(* Logix 5000 AddOnInstructionDefinition export SPEL_SpeedS; software revision 30.01 *)

ADD_ON_INSTRUCTION SPEL_ExecCmd   (* revision 1.2 *)
// Executes a command in the robot controller.  Normally this is called by higher level AOIs.
VAR_INPUT
   Start : BOOL; {required}
   MaxTime : DINT := 3000; {required}
END_VAR
VAR_OUTPUT
   InCycle : BOOL; {access Read Only, visible}
   Done : BOOL; {access Read Only, visible}
   Error : BOOL; {access Read Only, visible}
END_VAR
VAR_IN_OUT
   ExtInputs : AB:ETHERNET_MODULE_INT_128Bytes:I:0; {required}
        .DATA[0].0   // ExtCmdGet
        .DATA[0].1   // ExtRespSet
        .DATA[0].2   // ExtCmdResult
        .DATA[0].3   // ExtError
   ExtOutputs : AB:ETHERNET_MODULE_INT_128Bytes:O:0; {required}
        .DATA[0].0   // ExtCmdSet
        .DATA[0].1   // ExtRespGet
        .DATA[0].2   // ExtCmdReset
END_VAR
VAR_INPUT
   Cmd : INT; {required}
   CmdParam1 : INT; {required}
   CmdParam2 : INT; {required}
   CmdParam3 : INT; {required}
   CmdParam4 : INT; {required}
   CmdParam5 : INT; {required}
   CmdParam6 : INT; {required}
   CmdParam7 : INT; {required}
END_VAR
VAR_OUTPUT
   CmdEcho : INT; {access Read Only, visible}
   Resp1 : INT; {access Read Only, visible}
   Resp2 : INT; {access Read Only, visible}
   Resp3 : INT; {access Read Only, visible}
   Resp4 : INT; {access Read Only, visible}
   Resp5 : INT; {access Read Only, visible}
   Resp6 : INT; {access Read Only, visible}
   Resp7 : INT; {access Read Only, visible}
   ErrCode1 : INT; {access Read Only, visible}
   ErrCode2 : INT; {access Read Only, visible}
END_VAR
VAR
   ExtReset : BOOL; {access None}
   ExtError : BOOL; {access None}
   ExtCmdSet : BOOL; {access None}   // Cmd Ready
   ExtCmdGet : BOOL; {access None}   // Cmd Received
   CmdXferDone : BOOL; {access None}
   ExtRespSet : BOOL; {access None}   // Resp Ready
   RespXferDone : BOOL; {access None}
   ExtCmdResult : BOOL; {access None}   // Normal or Error?
   TmrCmdDataRdy : TIMER := (PRE := 5); {access None}
   OneShotDoneOff : BOOL; {access None}
   OneShotStart : BOOL; {access None}
   StartInit : BOOL; {access None}
   OneShotStartError : BOOL; {access None}
   TmrCycle : TIMER := (PRE := 5000); {access None}
   OneshotTmrPreset : BOOL; {access None}
   TmrCmdSet : TIMER := (PRE := 20); {access None}
   OnShotCmdDataXfer : BOOL; {access None}
   OneShotRespDataXfer : BOOL; {access None}
   OneShotDataRdy : BOOL; {access None}
   OtherCmdInCycle : BOOL; {access None}
   s : BOOL; {access None}
   OneShotUnsetCmdIncycle : BOOL; {access None}
   OneShotSetCmdIncycle : BOOL; {access None}
   OneShotSetOtherCmdInCycleError : BOOL; {access None}
   OneShotSetBit : BOOL; {access None}
   MaxTimeError : BOOL; {access None}
END_VAR

ROUTINE Logic   (* ladder *)
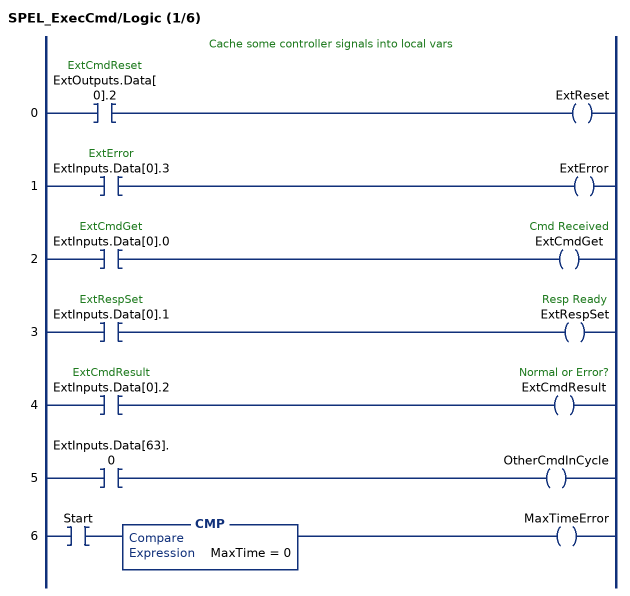
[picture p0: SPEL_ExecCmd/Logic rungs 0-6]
   // Cache some controller signals into local vars
   0: XIC(ExtOutputs.Data[0].2)OTE(ExtReset);
   1: XIC(ExtInputs.Data[0].3)OTE(ExtError);
   2: XIC(ExtInputs.Data[0].0)OTE(ExtCmdGet);
   3: XIC(ExtInputs.Data[0].1)OTE(ExtRespSet);
   4: XIC(ExtInputs.Data[0].2)OTE(ExtCmdResult);
   5: XIC(ExtInputs.Data[63].0)OTE(OtherCmdInCycle);
   6: XIC(Start)CMP(MaxTime = 0)OTE(MaxTimeError);
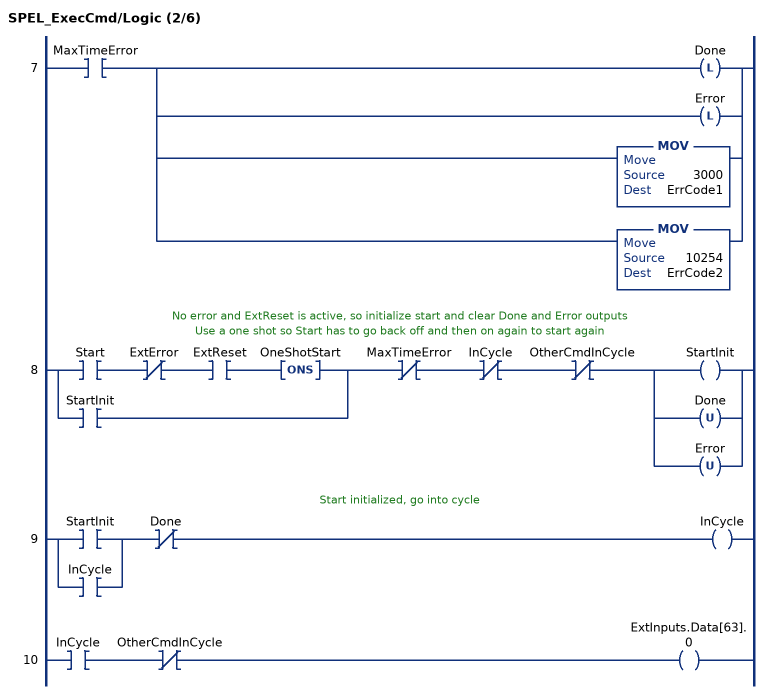
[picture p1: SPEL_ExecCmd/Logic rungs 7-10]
   7: XIC(MaxTimeError)[OTL(Done) ,OTL(Error) ,MOV(3000,ErrCode1) ,MOV(10254,ErrCode2) ];
   // No error and ExtReset is active, so initialize start and clear Done and Error outputs
   // Use a one shot so Start has to go back off and then on again to start again
   8: [XIC(Start) XIO(ExtError) XIC(ExtReset) ONS(OneShotStart) ,XIC(StartInit) ]XIO(MaxTimeError)XIO(InCycle)XIO(OtherCmdInCycle)[OTE(StartInit) ,OTU(Done) ,OTU(Error) ];
   // Start initialized, go into cycle
   9: [XIC(StartInit) ,XIC(InCycle) ]XIO(Done)OTE(InCycle);
   10: XIC(InCycle)XIO(OtherCmdInCycle)OTE(ExtInputs.Data[63].0);
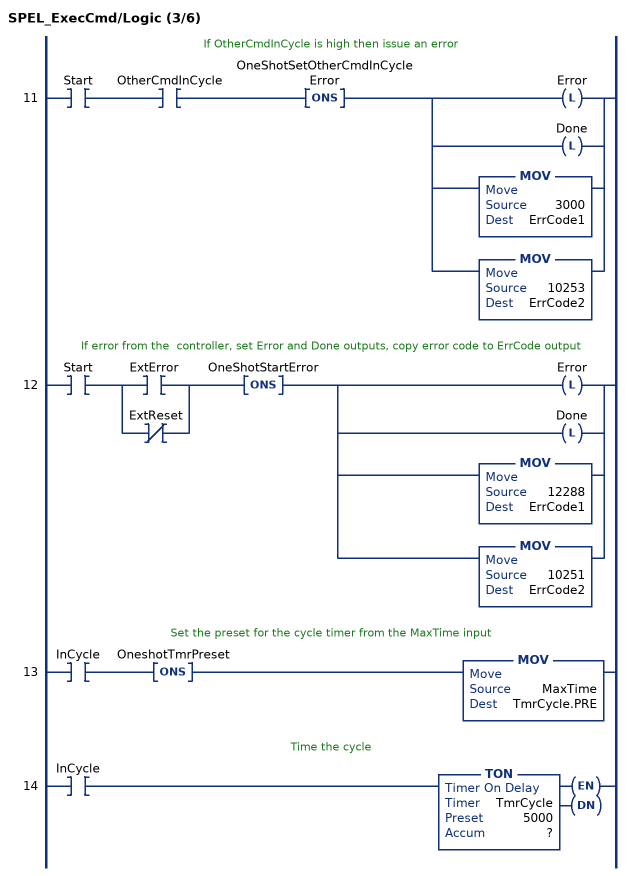
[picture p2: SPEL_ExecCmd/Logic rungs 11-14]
   // If OtherCmdInCycle is high then issue an error
   11: XIC(Start)XIC(OtherCmdInCycle)ONS(OneShotSetOtherCmdInCycleError)[OTL(Error) ,OTL(Done) ,MOV(3000,ErrCode1) ,MOV(10253,ErrCode2) ];
   // If error from the  controller, set Error and Done outputs, copy error code to ErrCode output
   12: XIC(Start)[XIC(ExtError) ,XIO(ExtReset) ]ONS(OneShotStartError)[OTL(Error) ,OTL(Done) ,MOV(12288,ErrCode1) ,MOV(10251,ErrCode2) ];
   // Set the preset for the cycle timer from the MaxTime input
   13: XIC(InCycle)ONS(OneshotTmrPreset)MOV(MaxTime,TmrCycle.PRE);
   // Time the cycle
   14: XIC(InCycle)TON(TmrCycle,?,?);
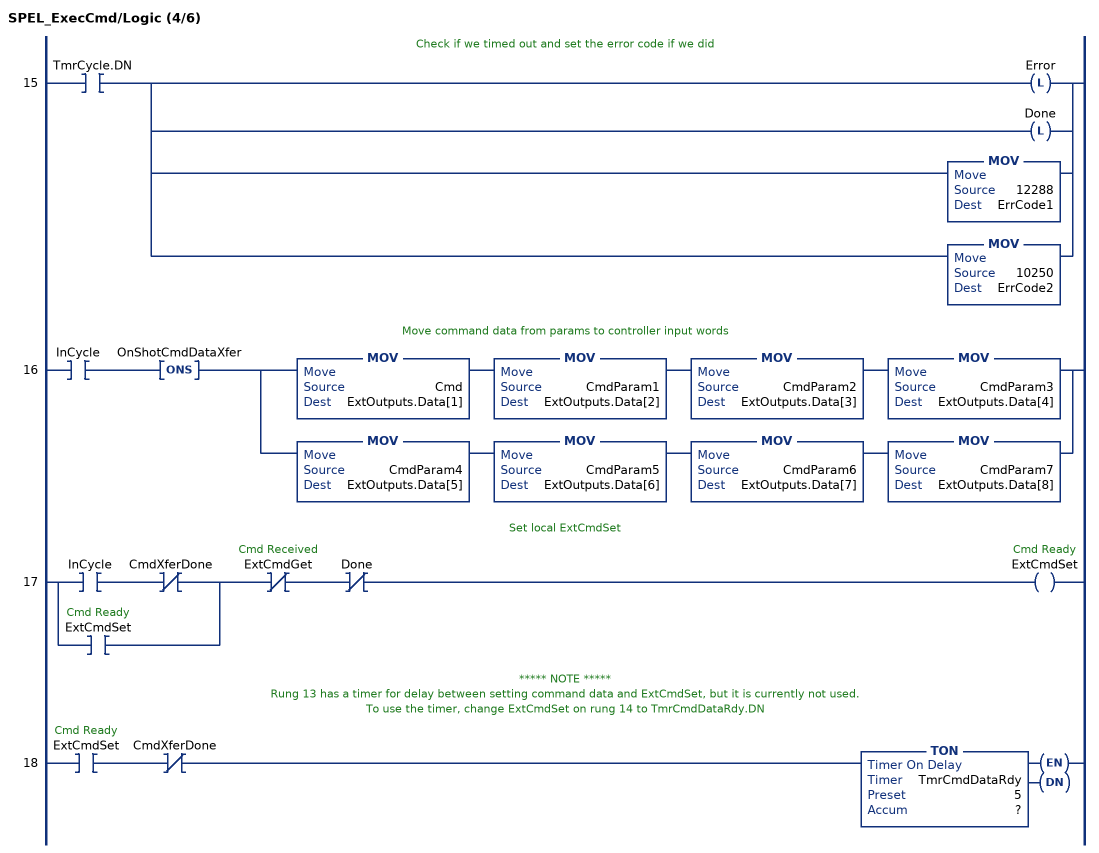
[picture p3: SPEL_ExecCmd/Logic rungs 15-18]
   // Check if we timed out and set the error code if we did
   15: XIC(TmrCycle.DN)[OTL(Error) ,OTL(Done) ,MOV(12288,ErrCode1) ,MOV(10250,ErrCode2) ];
   // Move command data from params to controller input words
   16: XIC(InCycle)ONS(OnShotCmdDataXfer)[MOV(Cmd,ExtOutputs.Data[1]) MOV(CmdParam1,ExtOutputs.Data[2]) MOV(CmdParam2,ExtOutputs.Data[3]) MOV(CmdParam3,ExtOutputs.Data[4]) ,MOV(CmdParam4,ExtOutputs.Data[5]) MOV(CmdParam5,ExtOutputs.Data[6]) MOV(CmdParam6,ExtOutputs.Data[7]) MOV(CmdParam7,ExtOutputs.Data[8]) ];
   // Set local ExtCmdSet
   17: [XIC(InCycle) XIO(CmdXferDone) ,XIC(ExtCmdSet) ]XIO(ExtCmdGet)XIO(Done)OTE(ExtCmdSet);
   // ***** NOTE *****
   // Rung 13 has a timer for delay between setting command data and ExtCmdSet, but it is currently not used.
   // To use the timer, change ExtCmdSet on rung 14 to TmrCmdDataRdy.DN
   18: XIC(ExtCmdSet)XIO(CmdXferDone)TON(TmrCmdDataRdy,?,?);
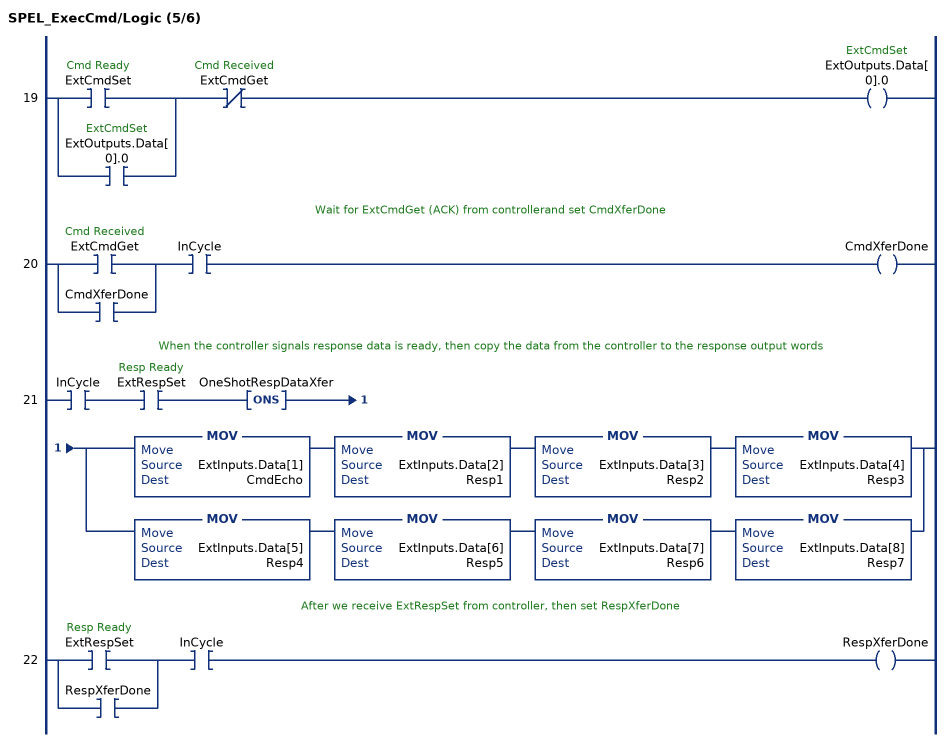
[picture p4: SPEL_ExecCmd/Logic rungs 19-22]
   19: [XIC(ExtCmdSet) ,XIC(ExtOutputs.Data[0].0) ]XIO(ExtCmdGet)OTE(ExtOutputs.Data[0].0);
   // Wait for ExtCmdGet (ACK) from controllerand set CmdXferDone
   20: [XIC(ExtCmdGet) ,XIC(CmdXferDone) ]XIC(InCycle)OTE(CmdXferDone);
   // When the controller signals response data is ready, then copy the data from the controller to the response output words
   21: XIC(InCycle)XIC(ExtRespSet)ONS(OneShotRespDataXfer)[MOV(ExtInputs.Data[1],CmdEcho) MOV(ExtInputs.Data[2],Resp1) MOV(ExtInputs.Data[3],Resp2) MOV(ExtInputs.Data[4],Resp3) ,MOV(ExtInputs.Data[5],Resp4) MOV(ExtInputs.Data[6],Resp5) MOV(ExtInputs.Data[7],Resp6) MOV(ExtInputs.Data[8],Resp7) ];
   // After we receive ExtRespSet from controller, then set RespXferDone
   22: [XIC(ExtRespSet) ,XIC(RespXferDone) ]XIC(InCycle)OTE(RespXferDone);
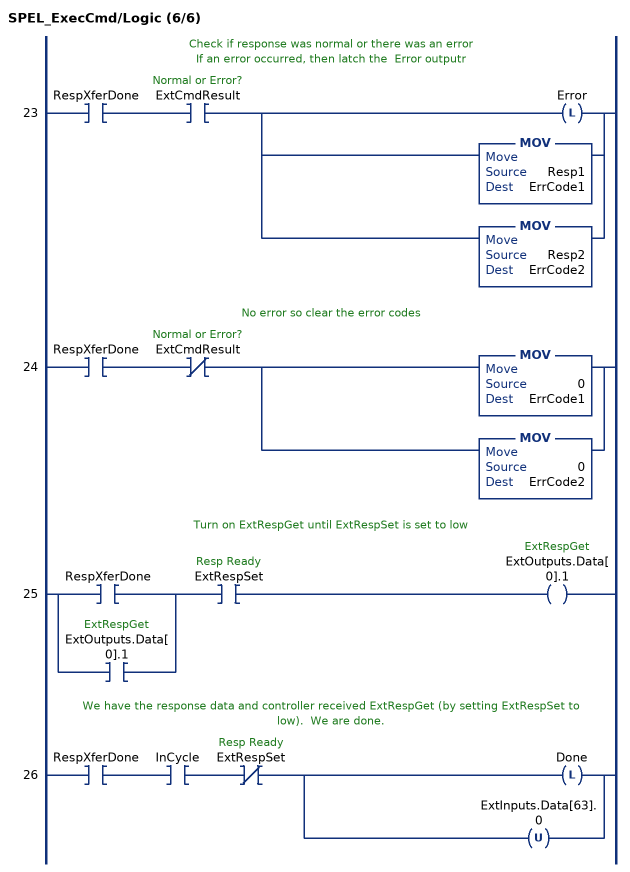
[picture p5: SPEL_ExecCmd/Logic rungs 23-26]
   // Check if response was normal or there was an error
   // If an error occurred, then latch the  Error outputr
   23: XIC(RespXferDone)XIC(ExtCmdResult)[OTL(Error) ,MOV(Resp1,ErrCode1) ,MOV(Resp2,ErrCode2) ];
   // No error so clear the error codes
   24: XIC(RespXferDone)XIO(ExtCmdResult)[MOV(0,ErrCode1) ,MOV(0,ErrCode2) ];
   // Turn on ExtRespGet until ExtRespSet is set to low
   25: [XIC(RespXferDone) ,XIC(ExtOutputs.Data[0].1) ]XIC(ExtRespSet)OTE(ExtOutputs.Data[0].1);
   // We have the response data and controller received ExtRespGet (by setting ExtRespSet to low).  We are done.
   26: XIC(RespXferDone)XIC(InCycle)XIO(ExtRespSet)[OTL(Done) ,OTU(ExtInputs.Data[63].0) ];
END_ROUTINE
END_ADD_ON_INSTRUCTION

ADD_ON_INSTRUCTION SPEL_SpeedS   (* revision 1.2, vendor SEIKO EPSON CORP. *)
// Sets the arm speed setting of CP motion. This will set the depart, and approach speed as well.
VAR_OUTPUT
   InCycle : BOOL; {access Read Only, visible}
   Done : BOOL; {access Read Only, visible}
   Error : BOOL; {access Read Only, visible}
END_VAR
VAR_INPUT
   Start : BOOL; {required}
   Speed : REAL; {required}
   ApproSpeed : REAL; {required}
   DepartSpeed : REAL; {required}
END_VAR
VAR_IN_OUT
   ExtInputs : AB:ETHERNET_MODULE_INT_128Bytes:I:0; {required}
   ExtOutputs : AB:ETHERNET_MODULE_INT_128Bytes:O:0; {required}
END_VAR
VAR_OUTPUT
   ErrCode1 : INT; {access Read Only, visible}
   ErrCode2 : INT; {access Read Only, visible}
END_VAR
VAR
   ExecSpeedS : SPEL_ExecCmd := (MaxTime := 3000); {access None}
   OneShotStart : BOOL; {access None}
   StartInit : BOOL; {access None}
   ApproachSp : DINT; {access None}
   Approachx1000 : DINT; {access None}
   DepartSp : DINT; {access None}
   Departx1000 : DINT; {access None}
   Approach_INTS : INT[2]; {access None}
   Depart_INTS : INT[2]; {access None}
   Speedx1000 : DINT; {access None}
   Speed_INTS : INT[2]; {access None}
   ExecTimeout : DINT; {access None}
END_VAR

ROUTINE Logic   (* ladder *)
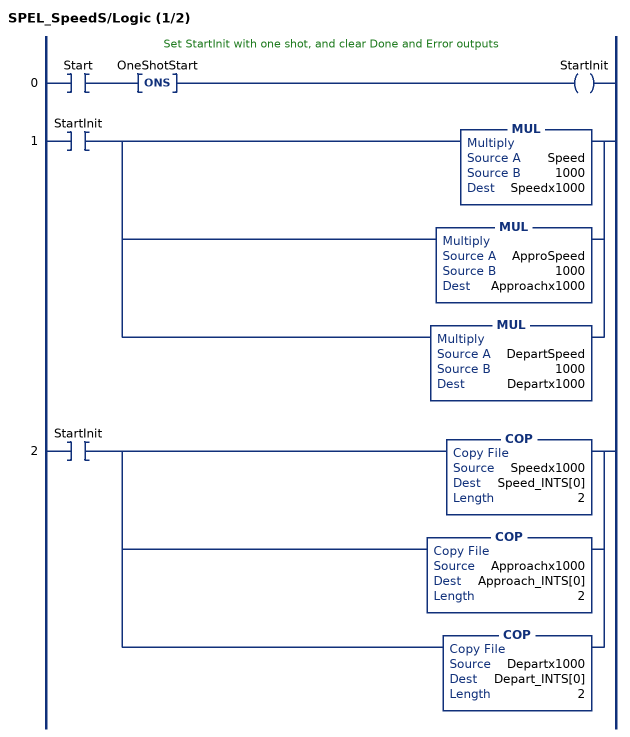
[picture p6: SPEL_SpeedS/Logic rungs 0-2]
   // Set StartInit with one shot, and clear Done and Error outputs
   0: XIC(Start)ONS(OneShotStart)OTE(StartInit);
   1: XIC(StartInit)[MUL(Speed,1000,Speedx1000) ,MUL(ApproSpeed,1000,Approachx1000) ,MUL(DepartSpeed,1000,Departx1000) ];
   2: XIC(StartInit)[COP(Speedx1000,Speed_INTS[0],2) ,COP(Approachx1000,Approach_INTS[0],2) ,COP(Departx1000,Depart_INTS[0],2) ];
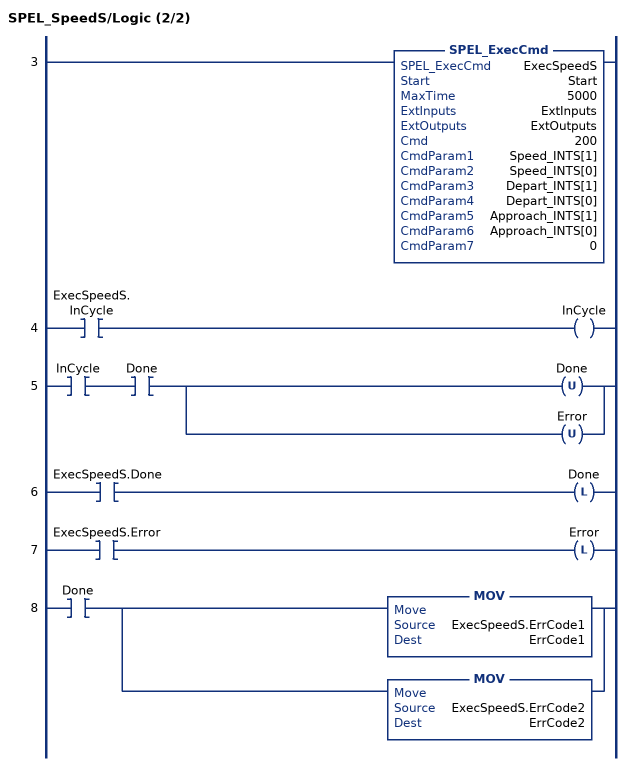
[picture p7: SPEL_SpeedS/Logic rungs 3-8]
   3: SPEL_ExecCmd(ExecSpeedS,Start,5000,ExtInputs,ExtOutputs,200,Speed_INTS[1],Speed_INTS[0],Depart_INTS[1],Depart_INTS[0],Approach_INTS[1],Approach_INTS[0],0);
   4: XIC(ExecSpeedS.InCycle)OTE(InCycle);
   5: XIC(InCycle)XIC(Done)[OTU(Done) ,OTU(Error) ];
   6: XIC(ExecSpeedS.Done)OTL(Done);
   7: XIC(ExecSpeedS.Error)OTL(Error);
   8: XIC(Done)[MOV(ExecSpeedS.ErrCode1,ErrCode1) ,MOV(ExecSpeedS.ErrCode2,ErrCode2) ];
END_ROUTINE
END_ADD_ON_INSTRUCTION
